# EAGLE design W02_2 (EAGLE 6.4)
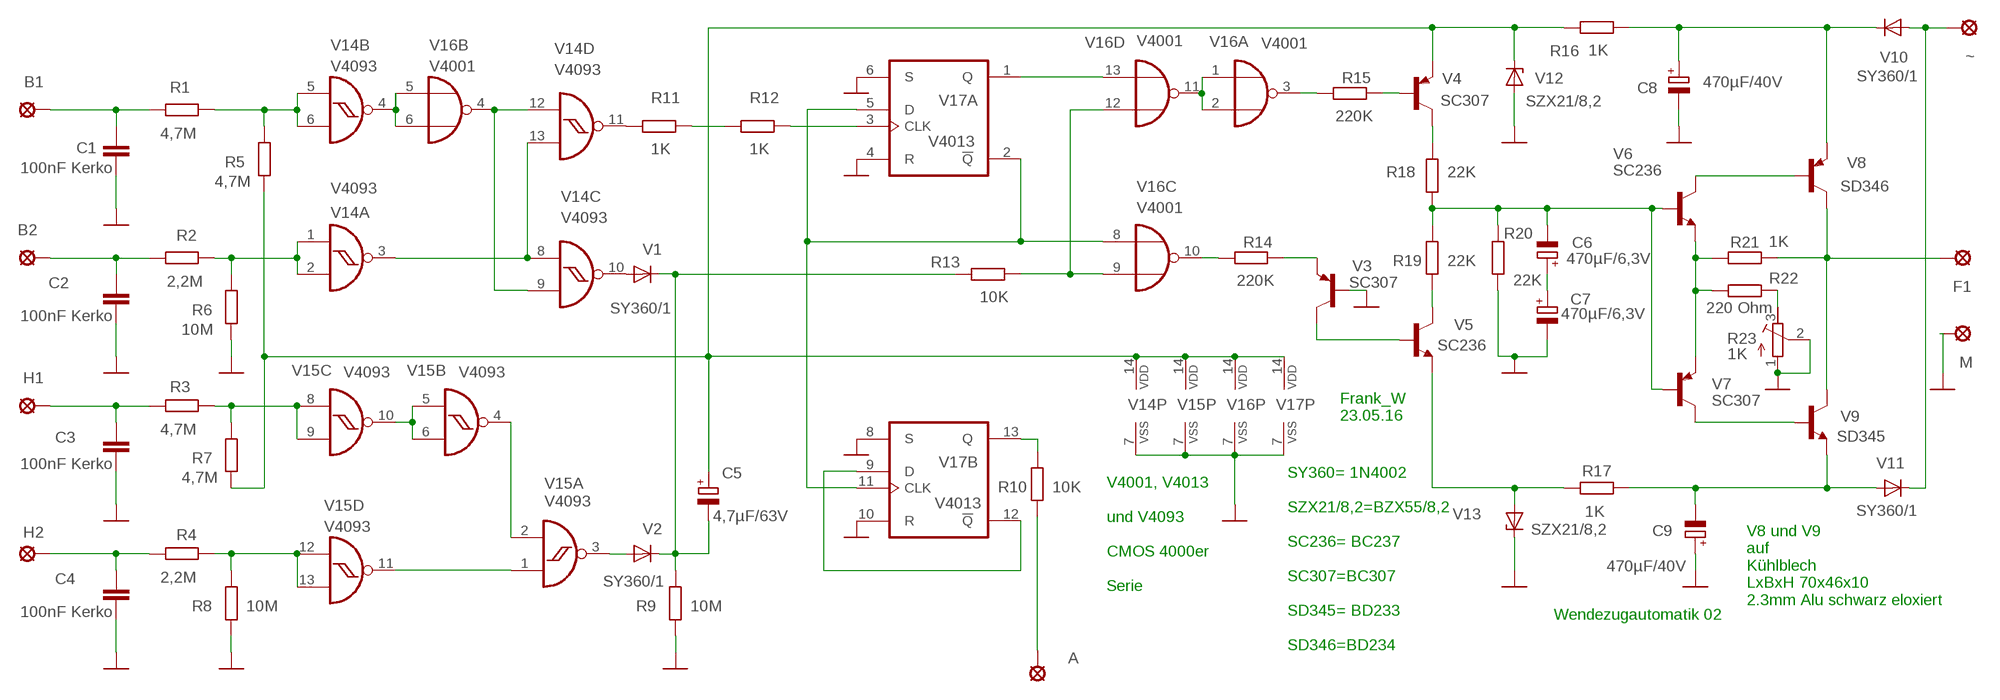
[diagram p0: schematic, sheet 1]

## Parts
A  LSP10  [LSP10]
B1  LSP10  [LSP10]
B2  LSP10  [LSP10]
C1  100nF Kerko  C-EU050-024X044  [C050-024X044]
C2  100nF Kerko  C-EU050-024X044  [C050-024X044]
C3  100nF Kerko  C-EU050-024X044  [C050-024X044]
C4  100nF Kerko  C-EU050-024X044  [C050-024X044]
C5  4,7µF/63V  CPOL-EUE5-5  [E5-5]
C6  470µF/6,3V  CPOL-EUE5-5  [E5-5]
C7  470µF/6,3V  CPOL-EUE5-5  [E5-5]
C8  470µF/40V  CPOL-EUE25-9AXIAL  [E25-9]
C9  470µF/40V  CPOL-EUE25-9AXIAL  [E25-9]
F1  LSP10  [LSP10]
H1  LSP10  [LSP10]
H2  LSP10  [LSP10]
M  LSP10  [LSP10]
R1  4,7M  R-EU_0207/12  [0207/12]
R2  2,2M  R-EU_0207/12  [0207/12]
R3  4,7M  R-EU_0207/12  [0207/12]
R4  2,2M  R-EU_0207/12  [0207/12]
R5  4,7M  R-EU_0207/12  [0207/12]
R6  10M  R-EU_0207/12  [0207/12]
R7  4,7M  R-EU_0207/12  [0207/12]
R8  10M  R-EU_0207/12  [0207/12]
R9  10M  R-EU_0207/12  [0207/12]
R10  10K  R-EU_0207/12  [0207/12]
R11  1K  R-EU_0207/12  [0207/12]
R12  1K  R-EU_0207/12  [0207/12]
R13  10K  R-EU_0207/12  [0207/12]
R14  220K  R-EU_0207/12  [0207/12]
R15  220K  R-EU_0207/12  [0207/12]
R16  1K  R-EU_0207/12  [0207/12]
R17  1K  R-EU_0207/12  [0207/12]
R18  22K  R-EU_0207/12  [0207/12]
R19  22K  R-EU_0207/12  [0207/12]
R20  22K  R-EU_0207/12  [0207/12]
R21  1K  R-EU_0207/12  [0207/12]
R22  220 Ohm  R-EU_0207/12  [0207/12]
R23  1K  R-TRIMM3296P  [RTRIM3296P]
V1  SY360/1  1N4004  [DO41-10]
V2  SY360/1  1N4004  [DO41-10]
V3  SC307  BC448  [TO92-EBC]
V4  SC307  BC307  [TO92]
V5  SC236  BC449  [TO92-EBC]
V6  SC236  BC449  [TO92-EBC]
V7  SC307  BC448  [TO92-EBC]
V8  SD346  BD140  [TO126]
V9  SD345  BD139  [TO126]
V10  SY360/1  1N4004  [DO41-10]
V11  SY360/1  1N4004  [DO41-10]
V12  SZX21/8,2  ZENER-DIODEZD-2.5  [ZDIO-2.5]
V13  SZX21/8,2  ZENER-DIODEZD-2.5  [ZDIO-2.5]
V14  V4093  4093N  [DIL14]
V15  V4093  4093N  [DIL14]
V16  V4001  4001N  [DIL14]
V17  V4013  4013N  [DIL14]
~  LSP10  [LSP10]

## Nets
GND: C1.2 C2.2 C3.2 C4.2 C7.- C8.- C9.+ M.MP R6.2 R8.2 R9.2 R20.2 R23.1(A) R23.2(S) V3.B V12.A V13.C V14.7(P:VSS) V15.7(P:VSS) V16.7(P:VSS) V17.4(A:R) V17.6(A:S) V17.7(P:VSS) V17.8(B:S) V17.10(B:R)
N$1: B1.MP C1.1 R1.1
N$2: V14.4(B:O) V16.5(B:I0) V16.6(B:I1)
N$3: B2.MP C2.1 R2.1
N$4: R3.2 R7.1 V15.8(C:I0) V15.9(C:I1)
N$5: V15.5(B:I0) V15.6(B:I1) V15.10(C:O)
N$6: V14.3(A:O) V14.8(C:I0) V14.13(D:I1)
N$7: V1.A V14.10(C:O)
N$8: R11.2 V14.11(D:O)
N$9: V10.A V11.C ~.MP
N$10: C3.1 H1.MP R3.1
N$11: R4.2 R8.1 V15.12(D:I0) V15.13(D:I1)
N$12: V14.9(C:I1) V14.12(D:I0) V16.4(B:O)
N$13: C4.1 H2.MP R4.1
N$14: V15.1(A:I0) V15.11(D:O)
N$15: V15.2(A:I1) V15.4(B:O)
N$16: C6.- R18.2 R19.1 R20.1 V6.B V7.B
N$17: V2.A V15.3(A:O)
N$18: C6.+ C7.+
N$19: R11.1 R12.2
N$20: R12.1 V17.3(A:CLK)
N$21: V16.8(C:I0) V17.2(A:!Q) V17.5(A:D) V17.11(B:CLK)
N$22: R22.2 R23.3(E)
N$23: C8.+ R16.1 V8.1(E) V10.C
N$24: V17.9(B:D) V17.12(B:!Q)
N$25: A.MP R10.2
N$26: R10.1 V17.13(B:Q)
N$27: V16.13(D:I1) V17.1(A:Q)
N$28: R13.1 V16.9(C:I1) V16.12(D:I0)
N$29: V16.1(A:I0) V16.2(A:I1) V16.11(D:O)
N$30: R15.2 V16.3(A:O)
N$31: R14.1 V3.E
N$32: R14.2 V16.10(C:O)
N$33: R15.1 V4.2(B)
N$34: R18.1 V4.3(C)
N$35: C5.- R9.1 R13.2 V1.C V2.C
N$36: R19.2 V5.C
N$37: V3.C V5.B
N$38: R21.2 R22.1 V6.E V7.E
N$39: V6.C V8.3(B)
N$40: F1.MP R21.1 V8.2(C) V9.2(C)
N$43: R1.2 R5.1 V14.5(B:I0) V14.6(B:I1)
N$44: V7.C V9.3(B)
N$45: R2.2 R6.1 V14.1(A:I0) V14.2(A:I1)
N$46: C9.- R17.2 V9.1(E) V11.A
N$47: R17.1 V5.E V13.A
N$48: C5.+ R5.2 R7.2 R16.2 V4.1(E) V12.C V14.14(P:VDD) V15.14(P:VDD) V16.14(P:VDD) V17.14(P:VDD)

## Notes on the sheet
- Frank_W
  23.05.16
- V4001, V4013
  
  und V4093
  
  CMOS 4000er
  
  Serie
- V8 und V9
  auf
  Kühlblech
  LxBxH 70x46x10
  2.3mm Alu schwarz eloxiert
- Wendezugautomatik 02
- SY360= 1N4002
  
  SZX21/8,2=BZX55/8,2
  
  SC236= BC237
  
  SC307=BC307
  
  SD345= BD233
  
  SD346=BD234

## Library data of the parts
A B1 B2 F1 H1 H2 M ~ = solpad:LSP10: SOLDER PAD
C1-C4 = rcl:C-EU: CAPACITOR, European symbol
C5-C9 = rcl:CPOL-EU: POLARIZED CAPACITOR, European symbol
R1-R22 = rcl:R-EU_: RESISTOR, European symbol
R23 = rcl:R-TRIMM: Trimm resistor
V1 V2 V10 V11 = diode:1N4004: DIODE
V3 V7 = transistor-pnp:BC448*: PNP Transistror
V4 = transistor-pnp:BC307: PNP Transistor
V5 V6 = transistor-npn:BC449*: NPN Transistor
V8 = transistor-pnp:BD140: PNP Transistor
V9 = transistor:BD139: NPN TRANSISTOR
V12 V13 = diode:ZENER-DIODE: Z-Diode
V14 V15 = 40xx:4093: Quad 2-input NAND schmitt trigger
V16 = 40xx:4001: Quad 2-input NOR
V17 = 40xx:4013: Dual D FLIP FLOP, set/reset

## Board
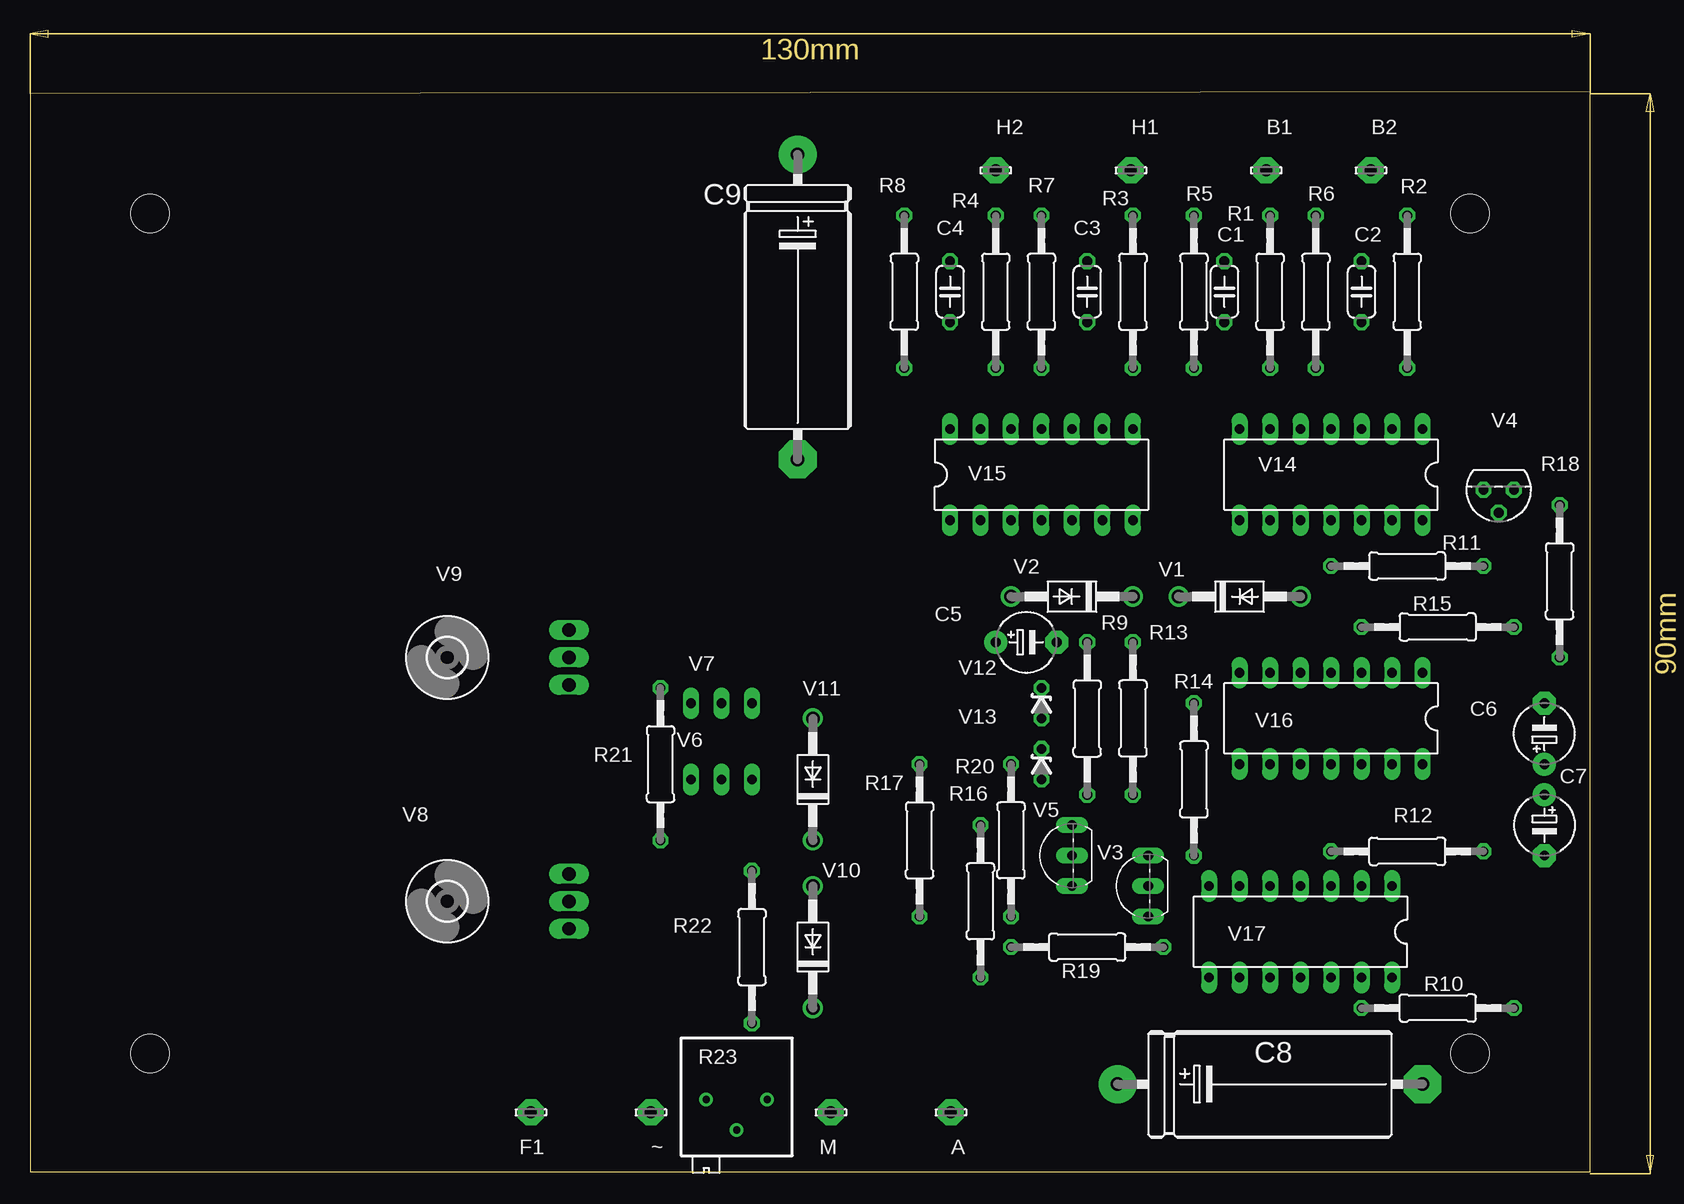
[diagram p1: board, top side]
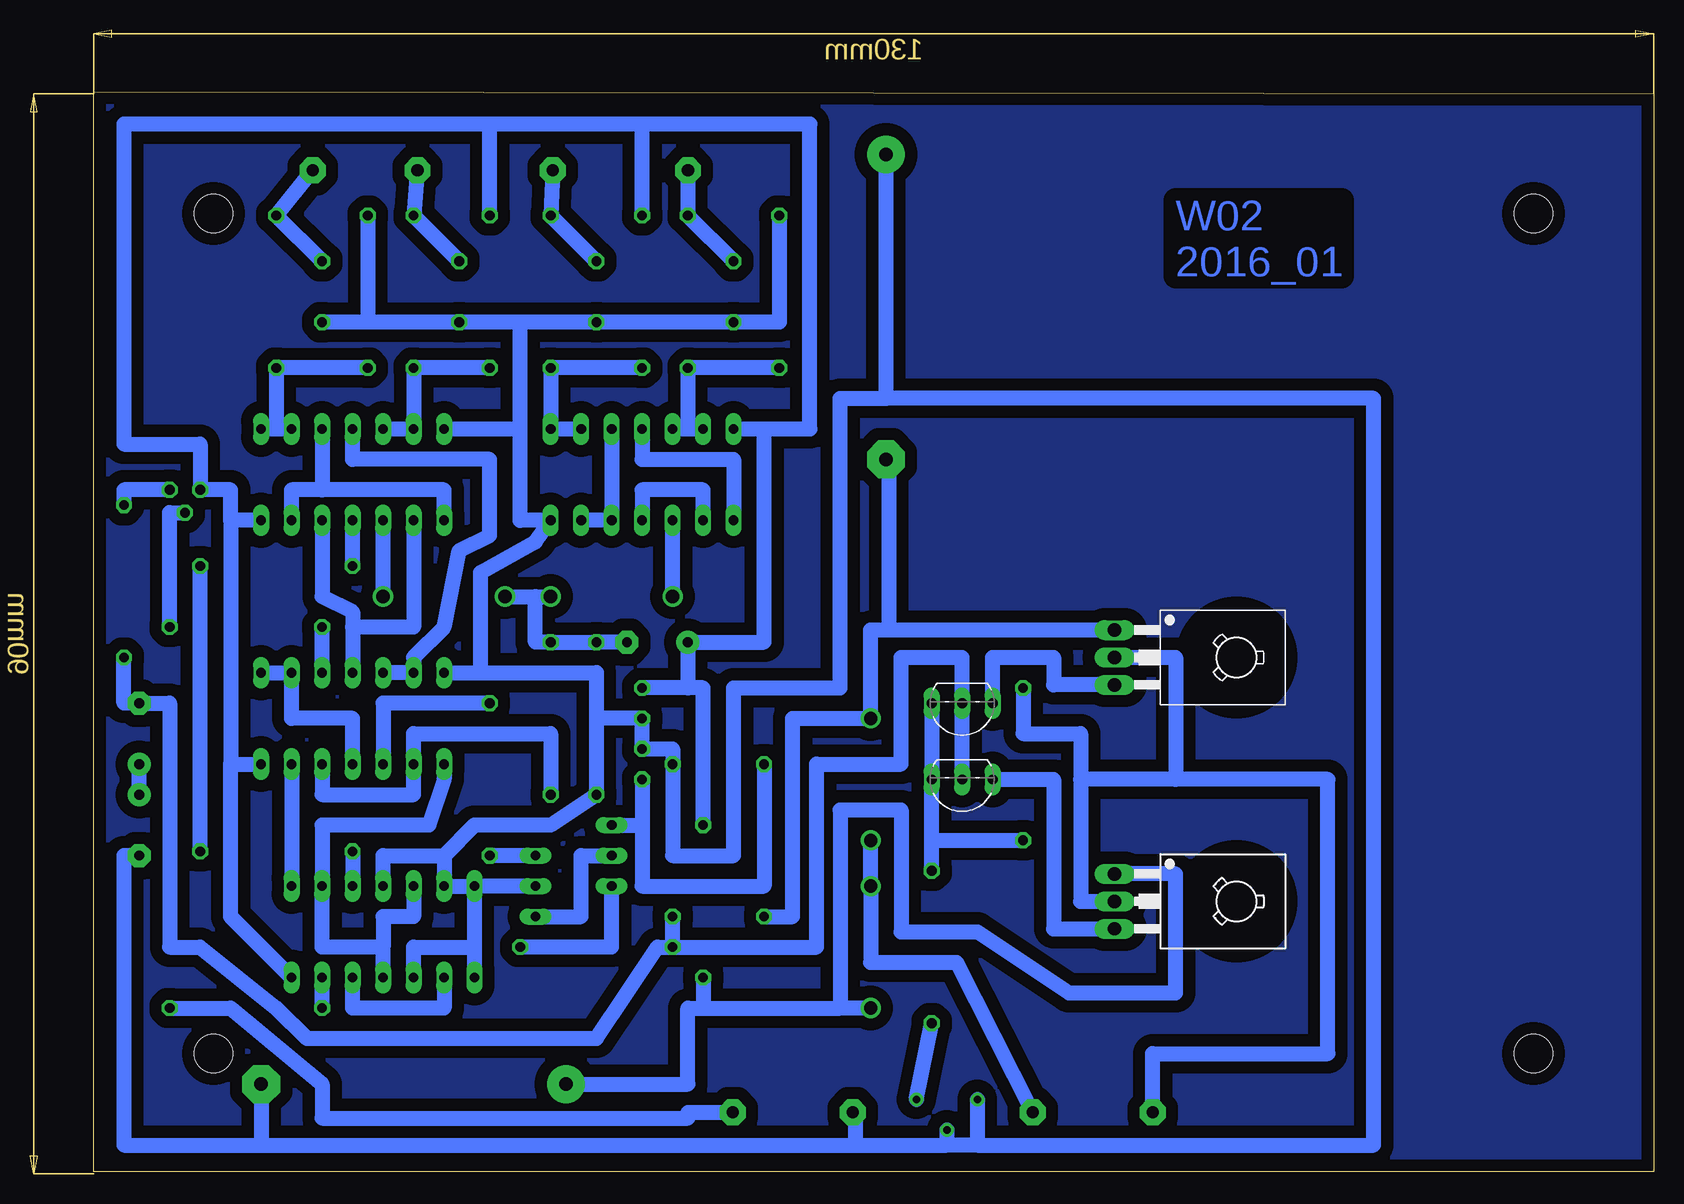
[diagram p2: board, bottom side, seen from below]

Size 135.3 x 95.3 mm. Coordinates in mm from the lower left corner, seen from the top.
Outline: 0,90 0,0.16 130,0.16 130,90.16 0,90
Copper layers (1*16): Top 0.035mm / dielectric 1.5mm / Bottom 0.035mm
Design rules "default *": minimum track width 20mil, minimum drill 24mil, track to track 8mil, track to pad 8mil, pad to pad 8mil, via to via 8mil, smd to smd 8mil, copper to edge 40mil, drill to drill 8mil, minimum pad ring 10mil, minimum via ring 8mil, stop-mask expansion 4mil, vias tented up to drill 0mil, thermal gap 20mil
Holes 3.2 mm at 120,10 10,10 10,80 120,80

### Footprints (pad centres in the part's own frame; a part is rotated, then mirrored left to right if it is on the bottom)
LSP10 = drill 1.016 pad 2.159 octagon: MP 0,0
C050-024X044 = drill 0.813 octagon: 1 -2.54,0; 2 2.54,0
E5-5 = drill 0.813 pad 1.905: + -2.54,0 | drill 0.813 pad 1.905 octagon: - 2.54,0
E25-9 = drill 1.118 pad 3.15: + -12.7,0 | drill 1.118 pad 3.15 octagon: - 12.7,0
0207/12 = drill 0.813 octagon: 1 -6.35,0; 2 6.35,0
RTRIM3296P = drill 0.61: 1 0,-2.54; 2 2.54,0; 3 0,2.54
3,2 = hole 3.2: 0,0
DO41-10 = drill 1.118: A 5.08,0; C -5.08,0
TO92-EBC = drill 0.813 long: B 0,-1.27; C -2.54,-1.27; E 2.54,-1.27
TO92 = drill 0.813 octagon: 1 1.27,0; 2 0,1.905; 3 -1.27,0
TO126 = drill 1.118 long: 1 -2.286,-5.08; 2 0,-5.08; 3 2.286,-5.08 | hole 3.302: 0,5.08
ZDIO-2.5 = drill 0.813 octagon: A 1.27,0; C -1.27,0
DIL14 = drill 0.813 long: 1 -7.62,-3.81; 2 -5.08,-3.81; 3 -2.54,-3.81; 4 0,-3.81; 5 2.54,-3.81; 6 5.08,-3.81; 7 7.62,-3.81; 8 7.62,3.81; 9 5.08,3.81; 10 2.54,3.81; 11 0,3.81; 12 -2.54,3.81; 13 -5.08,3.81; 14 -7.62,3.81

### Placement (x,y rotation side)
A  76.74,5.1 0 top
B1  103.01,83.6 0 top
B2  111.74,83.6 0 top
C1  99.53,73.49 270 top
C2  110.96,73.49 270 top
C3  88.1,73.49 270 top
C4  76.67,73.49 270 top
C5  83.02,44.28 0 top
C6  126.2,36.66 90 top
C7  126.2,29.04 270 top
C8  103.34,7.45 0 top
C9  63.97,72.22 270 top
F1  41.74,5.1 0 top
H1  91.74,83.6 0 top
H2  80.47,83.6 0 top
M  66.74,5.1 0 top
R1  103.34,73.49 270 top
R2  114.77,73.49 270 top
R3  91.91,73.49 270 top
R4  80.48,73.49 270 top
R5  96.99,73.49 90 top
R6  107.15,73.49 90 top
R7  84.29,73.49 90 top
R8  72.86,73.49 90 top
R9  88.1,37.93 270 top
R10  117.31,13.8 0 top
R11  114.77,50.63 180 top
R12  114.77,26.85 0 top
R13  91.91,37.93 90 top
R14  96.99,32.85 90 top
R15  117.31,45.55 180 top
R16  79.21,22.69 90 top
R17  74.13,27.77 270 top
R18  127.47,49.36 270 top
R19  88.1,18.88 0 top
R20  81.75,27.77 90 top
R21  52.54,34.12 270 top
R22  60.16,18.88 270 top
R23  58.89,6.18 270 top
U$2  [3,2]  34.76,43.01 0 top
U$3  [3,2]  34.76,22.69 0 top
V1  100.8,48.09 0 top
V2  86.83,48.09 180 top
V3  91.91,23.96 90 top
V4  122.39,56.98 180 top
V5  85.56,26.5 90 top
V6  57.62,31.58 180 bottom
V7  57.62,37.93 180 bottom
V8  39.84,22.69 270 bottom
V9  39.84,43.01 270 bottom
V10  65.24,18.88 90 top
V11  65.24,32.85 90 top
V12  84.29,39.2 270 top
V13  84.29,34.12 270 top
V14  108.42,58.25 180 top
V15  84.29,58.25 0 top
V16  108.42,37.93 180 top
V17  105.88,20.15 180 top
~  51.74,5.1 0 top

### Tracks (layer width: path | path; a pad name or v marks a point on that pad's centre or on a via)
GND
  Bottom 1.27: V14.7 94.45,62.06 | 94.45,62.06 94.45,70.95 | 94.45,70.95 C1.2 107.15,70.95 | 107.15,70.95 C2.2 | 94.45,70.95 C3.2 C4.2 72.86,70.95 R8.2 | R6.2 107.15,70.95 | 94.45,62.06 94.45,54.44 V15.7 93.18,52.64 97.74,50.1 97.74,41.74 | V16.7 97.74,41.74 | 97.74,41.74 88.1,41.74 88.1,37.93 | 88.1,37.93 R9.2 91.91,29.04 98.26,29.04 100.8,26.5 | V17.4 105.88,26.5 100.8,26.5 | V17.10 103.34,18.88 98.26,18.88 | 98.26,18.88 V17.8 | V17.7 V17.6 100.8,26.5 | V17.7 98.26,18.88 | C7.- 127.47,26.5 127.47,2.37 116.04,2.37 | 88.1,37.93 V12.A V13.C 81.75,35.39 R20.2 81.75,26.5 76.67,26.5 76.67,40.47 67.78,40.47 67.78,64.6 63.97,64.6 | C8.- 116.04,2.37 | R23.1 56.35,2.37 | 56.35,2.37 58.89,2.37 | V3.B V17.7 | 116.04,2.37 66.51,2.37 | 66.51,2.37 58.89,2.37 | 56.35,2.37 23.33,2.37 23.33,64.6 63.97,64.6 | C9.+ 63.97,64.6 | R23.2 58.89,2.37 | M.MP 66.51,5.1 66.51,2.37
N$1
  Bottom 1.27: C1.1 R1.1 B1.MP
N$2
  Bottom 1.27: V14.4 108.42,59.52 96.99,59.52 96.99,53.17 99.53,51.9 100.8,45.55 103.34,43.01 V16.6 V16.5
N$3
  Bottom 1.27: C2.1 R2.1 B2.MP
N$4
  Bottom 1.27: V15.9 V15.8 R3.2 R7.1
N$5
  Bottom 1.27: V15.10 V15.5 V15.6
N$6
  Bottom 1.27: V14.8 100.8,56.98 110.96,56.98 | 110.96,56.98 113.5,56.98 V14.13 | V14.3 110.96,56.98
N$7
  Bottom 1.27: V1.A V14.10
N$8
  Bottom 1.27: R11.2 V14.11
N$9
  Bottom 1.27: V11.C V10.A 65.24,17.61 58.09,17.61 ~.MP
N$10
  Bottom 1.27: H1.MP R3.1 C3.1
N$11
  Bottom 1.27: R8.1 R4.2 80.48,62.06 | V15.12 80.48,62.06 | 80.48,62.06 V15.13
N$12
  Bottom 1.27: V14.9 103.34,45.55 108.42,45.55 | V14.12 110.96,48.09 108.42,46.82 108.42,45.55 | 108.42,45.55 V16.4
N$13
  Bottom 1.27: H2.MP R4.1 C4.1
N$14
  Bottom 1.27: V15.11 84.29,59.52 76.67,59.52 V15.1
N$15
  Bottom 1.27: V15.2 79.21,56.98 84.29,56.98 V15.4
N$16
  Bottom 1.27: R18.2 127.47,39.2 C6.- 123.66,39.2 123.66,18.88 121.12,18.88 114.77,13.8 112.23,11.26 88.1,11.26 83.02,18.88 R19.1 | R19.1 69.74,18.88 69.74,34.12 62.7,34.12 62.7,43.01 57.62,43.01 V7.B V6.B | R19.1 R20.1
N$17
  Bottom 1.27: V2.A V15.3
N$18
  Bottom 1.27: C7.+ C6.+
N$19
  Bottom 1.27: R12.2 R11.1
N$20
  Bottom 1.27: R12.1 V17.3
N$21
  Bottom 1.27: V16.8 100.8,32.85 102.07,29.04 110.96,29.04 V17.2 110.96,18.88 105.88,18.88 | V17.11 105.88,18.88 | V17.5 103.34,21.42 105.88,21.42 105.88,18.88
N$22
  Bottom 1.27: R23.3 R22.2
N$23
  Bottom 1.27: C8.+ 80.48,7.45 80.48,13.8 79.21,13.8 | V10.C 67.78,13.8 | 67.78,13.8 67.78,30.31 62.7,30.31 62.7,20.15 56.35,20.15 48.73,15.07 39.84,15.07 39.84,24.98 V8.1 | 79.21,13.8 67.78,13.8 | R16.1 79.21,13.8
N$24
  Bottom 1.27: V17.9 100.8,13.8 108.42,13.8 V17.12
N$25
  Bottom 1.27: R10.2 118.58,13.8 110.96,7.45 110.96,4.62 80.48,4.62 80.48,5.1 A.MP
N$26
  Bottom 1.27: R10.1 V17.13
N$27
  Bottom 1.27: V16.13 V17.1
N$28
  Bottom 1.27: V16.12 110.96,31.58 103.34,31.58 V16.9 103.34,36.66 91.91,36.66 R13.1
N$29
  Bottom 1.27: V16.1 V16.2 113.5,37.93 108.42,37.93 V16.11
N$30
  Bottom 1.27: V16.3 R15.2
N$31
  Bottom 1.27: V3.E R14.1
N$32
  Bottom 1.27: R14.2 105.88,39.2 V16.10
N$33
  Bottom 1.27: R15.1 123.66,54.44 123.66,55.07 V4.2
N$34
  Bottom 1.27: V4.3 127.47,56.98 R18.1
N$35
  Bottom 1.27: V1.C 93.18,48.09 | 93.18,48.09 V2.C | C5.- R9.1 R13.2 93.18,44.28 93.18,48.09
N$36
  Bottom 1.27: R19.2 86.83,18.88 V5.C
N$37
  Bottom 1.27: V3.C 89.37,21.42 89.37,26.5 V5.B
N$38
  Bottom 1.27: R22.1 60.16,27.77 | 60.16,27.77 R21.2 | V7.E V6.E 60.16,27.77
N$39
  Bottom 1.27: V6.C 50,32.85 50,20.4 V8.3
N$40
  Bottom 1.27: 39.84,32.85 27.14,32.85 27.14,9.99 41.74,9.99 F1.MP | 39.84,32.85 47.74,32.85 | 47.74,32.85 47.74,22.69 V8.2 | R21.1 52.54,36.66 47.74,36.66 47.74,32.85 | V9.2 39.84,43.01 39.84,32.85
N$41
  pour Bottom (isolate 1.016): 0.47,90 130.01,90 130.01,-0.17 0.47,-0.17
N$43
  Bottom 1.27: R5.1 R1.2 V14.6 V14.5
N$44
  Bottom 1.27: V7.C 55.08,43.01 50,43.01 50,40.72 V9.3
N$45
  Bottom 1.27: R6.1 R2.2 114.77,62.06 | V14.1 114.77,62.06 | 114.77,62.06 V14.2
N$46
  Bottom 1.27: R17.2 71.74,21.42 71.74,37.93 V11.A 65.24,45.3 63.74,45.3 | V9.1 63.74,45.3 | C9.- 63.74,59.52 63.74,45.3
N$47
  Bottom 1.27: R17.1 74.13,23.96 84.29,23.96 84.29,29.04 | V5.E 84.29,29.04 | V13.A 84.29,29.04
N$48
  Bottom 1.27: V15.14 74.13,62.06 | 74.13,62.06 70.32,62.06 70.32,87.46 84.29,87.46 | 84.29,87.46 96.99,87.46 | 96.99,87.46 127.47,87.46 127.47,60.79 121.12,60.79 V4.1 118.58,56.98 118.58,54.44 | R5.2 96.99,87.46 | R7.2 84.29,87.46 | V14.14 118.58,54.44 | 118.58,54.44 118.58,34.12 | 118.58,34.12 V16.14 | V17.14 118.58,21.42 118.58,34.12 | R16.2 79.21,40.47 80.48,40.47 | 80.48,40.47 V12.C | 74.13,62.06 74.13,44.28 C5.+ 80.48,40.47

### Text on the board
Bottom: W02 / 2016_01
